(* Logix 5000 AddOnInstructionDefinition export Banner_QS18COD_Param_v4; software revision 33.00 *)

TYPE Banner_IOL_Port_v4 :   // UDT that has all of the data items necessary to communicate with a specific Port on a IO-Link Master
STRUCT
   Port_Controlled : INT;   // Each bit represents a port on an IO-Link Master. Set to 1 to tell AOI to control that port.
   Port_Activate : INT;   // Each bit represents a port on an IO-Link Master. When ON that port will process any commands in queue.
   Port_Read : INT;   // Each bit represents a port on an IO-Link Master. Used to determine when device AOI has requested a Read command.
   Port_Write : INT;   // Each bit represents a port on an IO-Link Master. Used to determine when device AOI has requested a Write command.
   Port_RW_Complete : INT;   // Each bit represents a port on an IO-Link Master. Tells device AOI that Read or Write request has been completed.
   Port_Device_Read : INT;
   Data_Transfer : SINT[190];   // Array to transfer data from IO-Master to device AOIs.
END_STRUCT
END_TYPE

TYPE Banner_QS18COD_RD_v4 :   // UDT that stores the Write Data for a QS18COD.
STRUCT
   Master_Cycle_Time : INT;
   Min_Cycle_Time : INT;
   M_Sequence_Capability : INT;
   IO_Link_Version_ID : INT;
   Process_Data_Input_Length : INT;
   Process_Data_Output_Length : INT;
   Combined_Vendor_ID : DINT;   // IO-Link Vendor ID
   Vendor_ID1 : INT;
   Vendor_ID2 : INT;
   Combined_Device_ID : DINT;   // IO-Link Device ID
   Device_ID1 : INT;
   Device_ID2 : INT;
   Device_ID3 : INT;
   Serial_Number : STRING;
   Quality_of_Health : INT;
   Normalized_Signal_Strength : INT;
   Quality_of_Teach : INT;
   Health_Lower_Limit : INT;
   Health_Upper_Limit : INT;
   Lower_Sensing_Threshold : INT;
   Upper_Sensing_Threshold : INT;
   Sensor_Operationl_Mode : INT;
END_STRUCT
END_TYPE

TYPE Banner_QS18COD_v4 :   // All of the parameters for a QS18COD.
STRUCT
   Initial_Global_Read : BOOL;   // Determines if all of the IO-Link data has been read into the PLC yet
   Command : INT;   // Value placed in here will activate a read or write to a specifc IO-Link Index
   Read_Data : Banner_QS18COD_RD_v4;   // Read Only Data
   Write_Data : Banner_QS18COD_WD_v4;   // Write Data
   Archive : Banner_QS18COD_WD_v4;   // Archive Data
   Reset : BOOL;   // Resets AOI. This will force a complete parameter read of the sensor.
END_STRUCT
END_TYPE

TYPE Banner_QS18COD_WD_v4 :   // UDT that stores the Write Data for a QS18COD.
STRUCT
   System_Command : INT;   // See IODD file for list of commands that can be activated via the System Command interface
   Parameter_Access_Lock : SINT;   // Write access to all parameters is prohibited while value is 1. Only this parameter can be adjusted when value is 1.
   Data_Storage_Lock : SINT;   // Automatic data storage is disabled when this value is equal to 1. Read access is not affected.
   Local_Parameterization_Lock : SINT;   // Parameterization via local control elements on device is disabled.
   Local_User_Interface_Lock : SINT;   // Operation of local user interface is disabled.
   BDC1_Switchpoint_Logic : INT;   // 0 = Light Operate, 1 = Dark Operate
   BDC1_BDC_Mode : INT;   // 1 = 1-Pt BGS, 128 = 2-Pt, 129 = Dynamic, 130 = Window or FGS, 131 = Dual
   BDC1_Hysteresis : DINT;   // Should always be 0
   User_Health_Setting : INT;   // 0 to 90
   Health_Mode : INT;   // 0=Auto, 1=User
   Threshold_Offset : INT;   // 0=8, 1=16, 2=32. Controls the Sensitivity of the Sensor.
   Auto_Compensaton : INT;   // 0=Disabled, 1=Enabled
   Delay_Timer_2 : DINT;   // 0 to 90000 ms
   Delay_Timer_1 : DINT;   // 0 to 90000 ms
   Delay_Mode : INT;   // 0=Disabled, 1=On Off Delay, 2=On One Shot, 3=Off One Shot
   Pin_2_Configuration : SINT;   // 0=Deactivated, 1=Emitter Enable, 2=Emitter Disabled, 3=Remote Input, 4=Detection Output, 5=Complimentary Output, 6=Health Output Active, 7=Health Output Inactive
   Polarity_of_Pins_2_and_4 : INT;   // 0 = Push Pull, 1 = PNP, 2 = NPN
END_STRUCT
END_TYPE

ADD_ON_INSTRUCTION Banner_QS18COD_Param_v4   (* revision 4.0, vendor Banner Engineering *)
// AOI to read and write parameter data to an IO-Link QS18 COD.
VAR_IN_OUT
   QS18COD : Banner_QS18COD_v4; {required}
   Port_Data : Banner_IOL_Port_v4; {required}
END_VAR
VAR_INPUT
   Port : DINT; {required}
END_VAR
VAR
   Local_Control : DINT; {access None}
   Global_Read_Command_Value : INT; {access None}
   Global_Write_Command_Value : INT; {access None}
   Command_Being_Processed : BOOL; {access None}
   Update_Archive : BOOL; {access None}
   Index_Write_Inprocess : INT; {access None}
   Index_Write_Control : INT; {access None}
   Inprocess_Index : DINT; {access None}
END_VAR

ROUTINE Logic   (* ladder *)
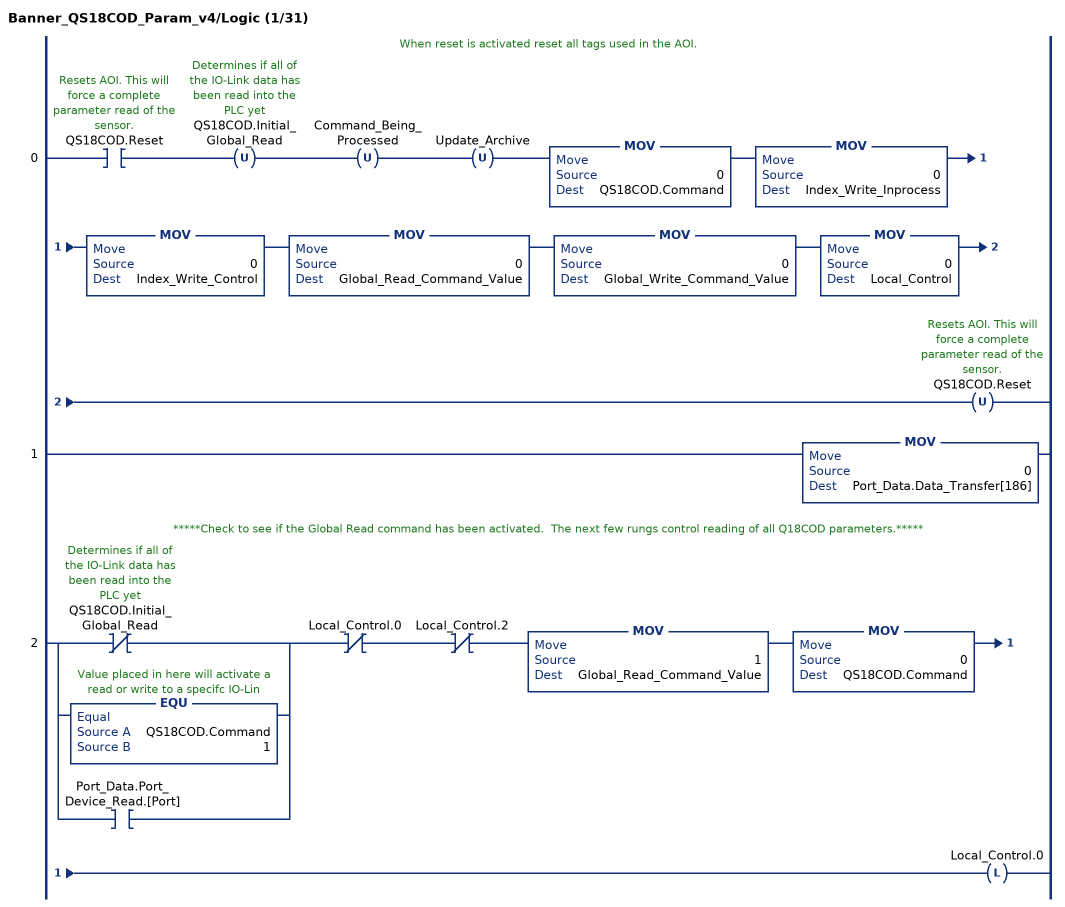
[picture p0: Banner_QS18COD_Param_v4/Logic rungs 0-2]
   // When reset is activated reset all tags used in the AOI.
   0: XIC(QS18COD.Reset)OTU(QS18COD.Initial_Global_Read)OTU(Command_Being_Processed)OTU(Update_Archive)MOV(0,QS18COD.Command)MOV(0,Index_Write_Inprocess)MOV(0,Index_Write_Control)MOV(0,Global_Read_Command_Value)MOV(0,Global_Write_Command_Value)MOV(0,Local_Control)OTU(QS18COD.Reset);
   1: MOV(0,Port_Data.Data_Transfer[186]);
   // *****Check to see if the Global Read command has been activated.  The next few rungs control reading of all Q18COD parameters.*****
   2: [XIO(QS18COD.Initial_Global_Read) ,EQU(QS18COD.Command,1) ,XIC(Port_Data.Port_Device_Read.[Port]) ]XIO(Local_Control.0)XIO(Local_Control.2)MOV(1,Global_Read_Command_Value)MOV(0,QS18COD.Command)OTL(Local_Control.0);
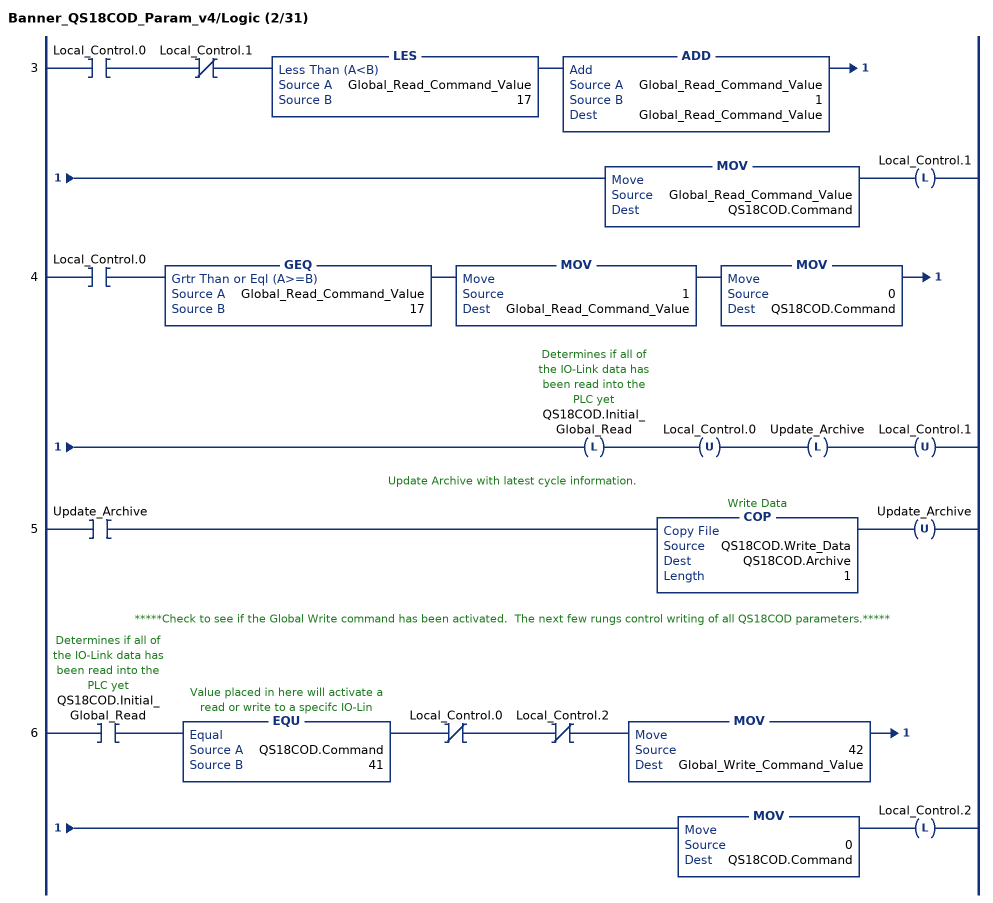
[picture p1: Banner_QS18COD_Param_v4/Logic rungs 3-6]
   3: XIC(Local_Control.0)XIO(Local_Control.1)LES(Global_Read_Command_Value,17)ADD(Global_Read_Command_Value,1,Global_Read_Command_Value)MOV(Global_Read_Command_Value,QS18COD.Command)OTL(Local_Control.1);
   4: XIC(Local_Control.0)GEQ(Global_Read_Command_Value,17)MOV(1,Global_Read_Command_Value)MOV(0,QS18COD.Command)OTL(QS18COD.Initial_Global_Read)OTU(Local_Control.0)OTL(Update_Archive)OTU(Local_Control.1);
   // Update Archive with latest cycle information.
   5: XIC(Update_Archive)COP(QS18COD.Write_Data,QS18COD.Archive,1)OTU(Update_Archive);
   // *****Check to see if the Global Write command has been activated.  The next few rungs control writing of all QS18COD parameters.*****
   6: XIC(QS18COD.Initial_Global_Read)EQU(QS18COD.Command,41)XIO(Local_Control.0)XIO(Local_Control.2)MOV(42,Global_Write_Command_Value)MOV(0,QS18COD.Command)OTL(Local_Control.2);
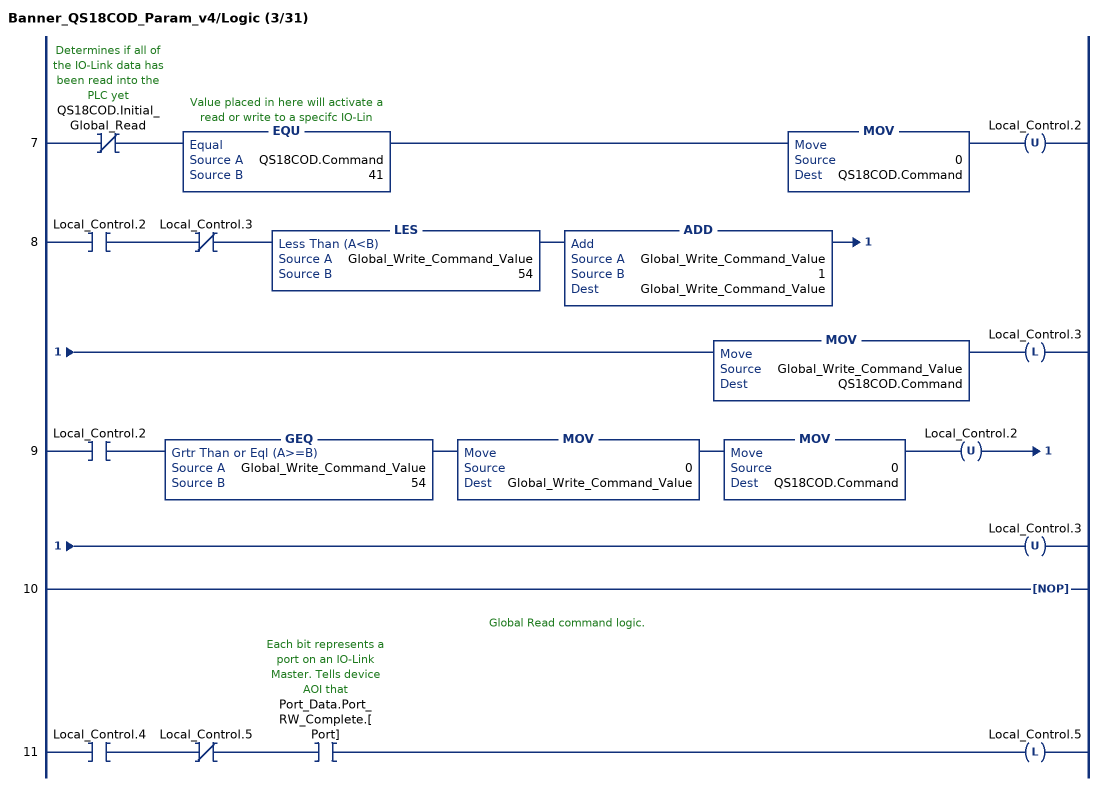
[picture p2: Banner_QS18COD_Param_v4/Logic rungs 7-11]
   7: XIO(QS18COD.Initial_Global_Read)EQU(QS18COD.Command,41)MOV(0,QS18COD.Command)OTU(Local_Control.2);
   8: XIC(Local_Control.2)XIO(Local_Control.3)LES(Global_Write_Command_Value,54)ADD(Global_Write_Command_Value,1,Global_Write_Command_Value)MOV(Global_Write_Command_Value,QS18COD.Command)OTL(Local_Control.3);
   9: XIC(Local_Control.2)GEQ(Global_Write_Command_Value,54)MOV(0,Global_Write_Command_Value)MOV(0,QS18COD.Command)OTU(Local_Control.2)OTU(Local_Control.3);
   10: NOP();
   // Global Read command logic.
   11: XIC(Local_Control.4)XIO(Local_Control.5)XIC(Port_Data.Port_RW_Complete.[Port])OTL(Local_Control.5);
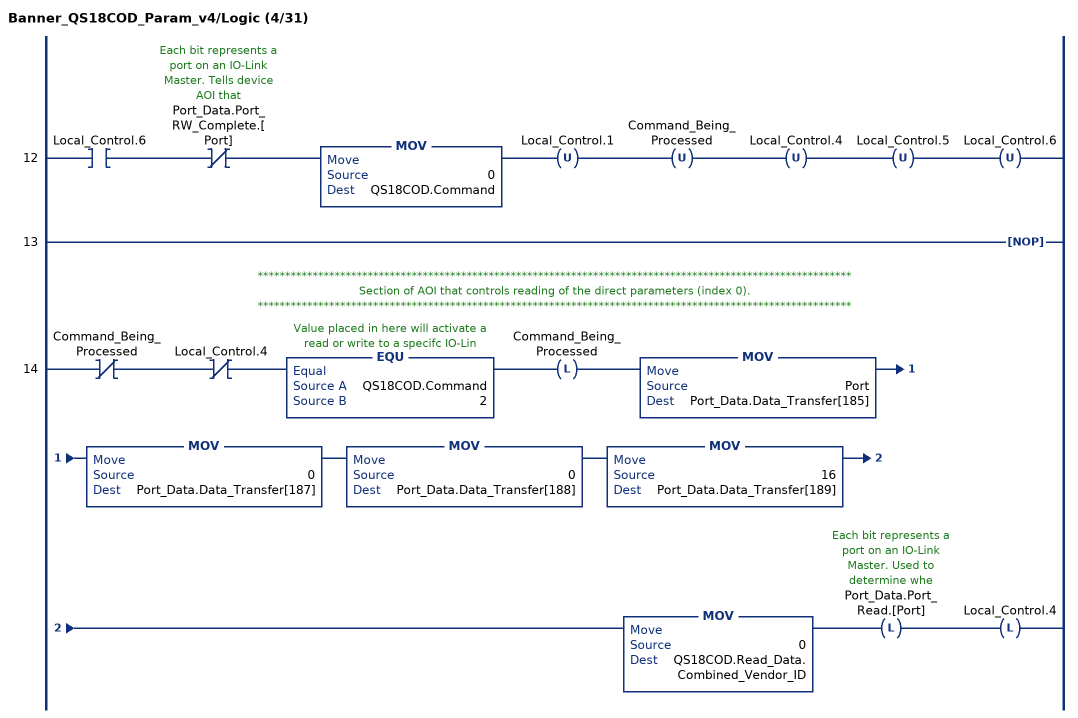
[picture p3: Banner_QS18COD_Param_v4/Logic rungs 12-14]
   12: XIC(Local_Control.6)XIO(Port_Data.Port_RW_Complete.[Port])MOV(0,QS18COD.Command)OTU(Local_Control.1)OTU(Command_Being_Processed)OTU(Local_Control.4)OTU(Local_Control.5)OTU(Local_Control.6);
   13: NOP();
   // ************************************************************************************************************
   // Section of AOI that controls reading of the direct parameters (index 0).
   // ************************************************************************************************************
   14: XIO(Command_Being_Processed)XIO(Local_Control.4)EQU(QS18COD.Command,2)OTL(Command_Being_Processed)MOV(Port,Port_Data.Data_Transfer[185])MOV(0,Port_Data.Data_Transfer[187])MOV(0,Port_Data.Data_Transfer[188])MOV(16,Port_Data.Data_Transfer[189])MOV(0,QS18COD.Read_Data.Combined_Vendor_ID)OTL(Port_Data.Port_Read.[Port])OTL(Local_Control.4);
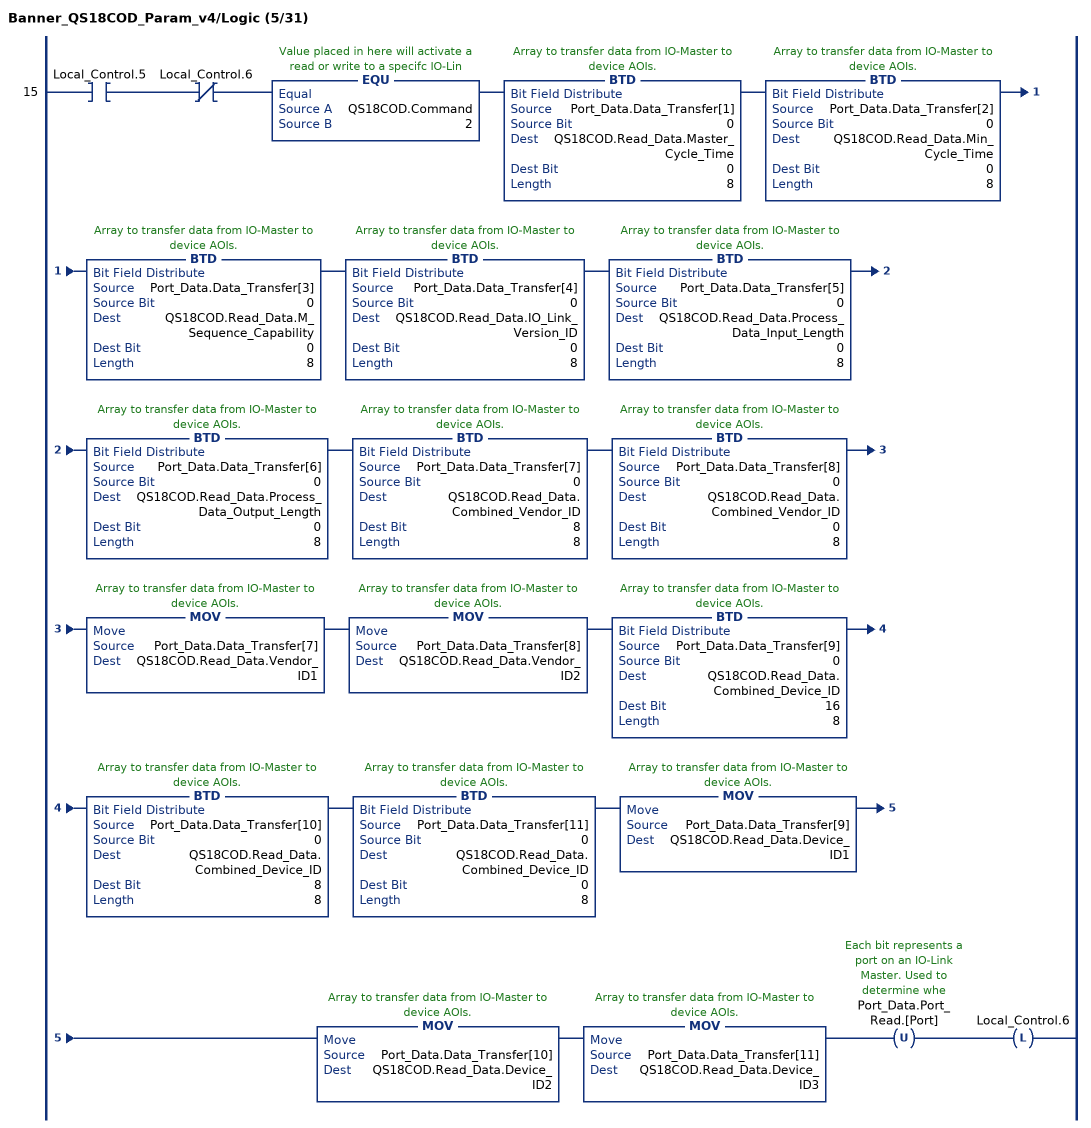
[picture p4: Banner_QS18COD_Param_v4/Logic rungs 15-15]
   15: XIC(Local_Control.5)XIO(Local_Control.6)EQU(QS18COD.Command,2)BTD(Port_Data.Data_Transfer[1],0,QS18COD.Read_Data.Master_Cycle_Time,0,8)BTD(Port_Data.Data_Transfer[2],0,QS18COD.Read_Data.Min_Cycle_Time,0,8)BTD(Port_Data.Data_Transfer[3],0,QS18COD.Read_Data.M_Sequence_Capability,0,8)BTD(Port_Data.Data_Transfer[4],0,QS18COD.Read_Data.IO_Link_Version_ID,0,8)BTD(Port_Data.Data_Transfer[5],0,QS18COD.Read_Data.Process_Data_Input_Length,0,8)BTD(Port_Data.Data_Transfer[6],0,QS18COD.Read_Data.Process_Data_Output_Length,0,8)BTD(Port_Data.Data_Transfer[7],0,QS18COD.Read_Data.Combined_Vendor_ID,8,8)BTD(Port_Data.Data_Transfer[8],0,QS18COD.Read_Data.Combined_Vendor_ID,0,8)MOV(Port_Data.Data_Transfer[7],QS18COD.Read_Data.Vendor_ID1)MOV(Port_Data.Data_Transfer[8],QS18COD.Read_Data.Vendor_ID2)BTD(Port_Data.Data_Transfer[9],0,QS18COD.Read_Data.Combined_Device_ID,16,8)BTD(Port_Data.Data_Transfer[10],0,QS18COD.Read_Data.Combined_Device_ID,8,8)BTD(Port_Data.Data_Transfer[11],0,QS18COD.Read_Data.Combined_Device_ID,0,8)MOV(Port_Data.Data_Transfer[9],QS18COD.Read_Data.Device_ID1)MOV(Port_Data.Data_Transfer[10],QS18COD.Read_Data.Device_ID2)MOV(Port_Data.Data_Transfer[11],QS18COD.Read_Data.Device_ID3)OTU(Port_Data.Port_Read.[Port])OTL(Local_Control.6);
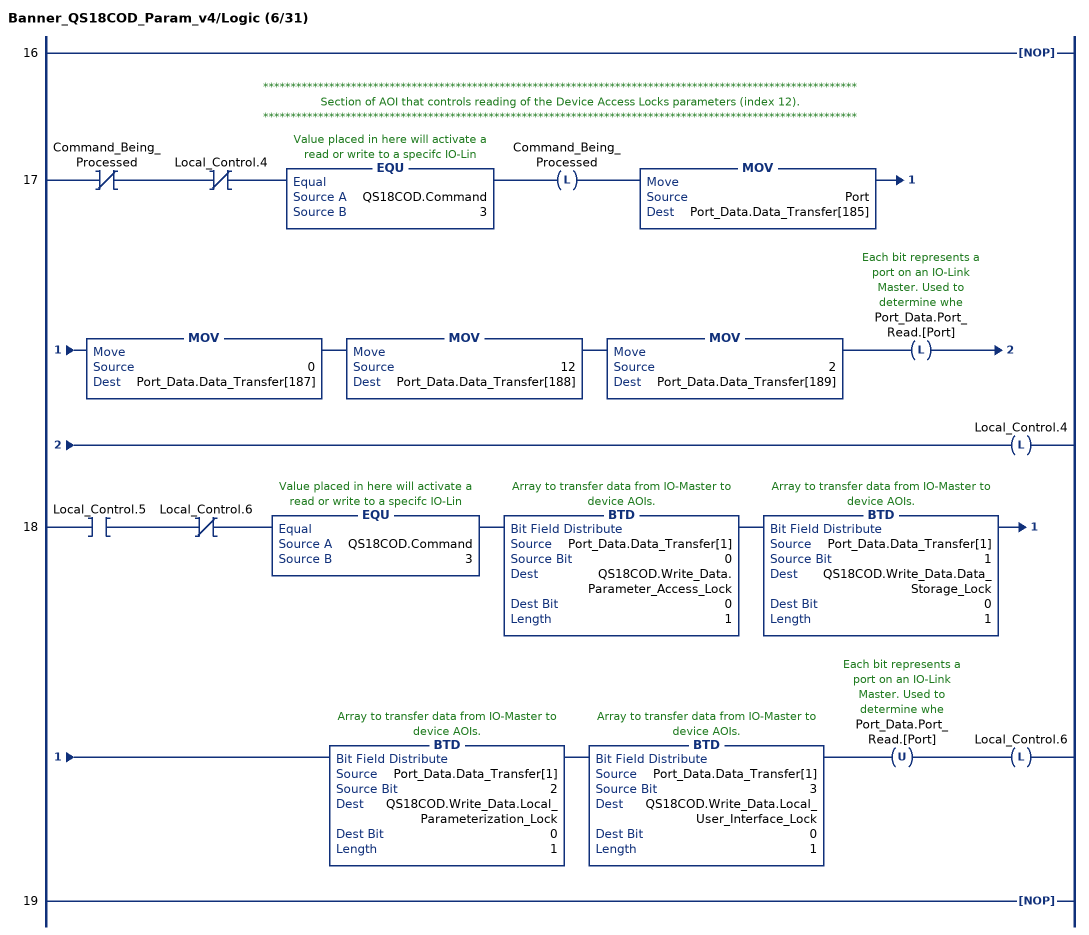
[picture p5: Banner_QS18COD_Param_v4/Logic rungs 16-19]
   16: NOP();
   // ************************************************************************************************************
   // Section of AOI that controls reading of the Device Access Locks parameters (index 12).
   // ************************************************************************************************************
   17: XIO(Command_Being_Processed)XIO(Local_Control.4)EQU(QS18COD.Command,3)OTL(Command_Being_Processed)MOV(Port,Port_Data.Data_Transfer[185])MOV(0,Port_Data.Data_Transfer[187])MOV(12,Port_Data.Data_Transfer[188])MOV(2,Port_Data.Data_Transfer[189])OTL(Port_Data.Port_Read.[Port])OTL(Local_Control.4);
   18: XIC(Local_Control.5)XIO(Local_Control.6)EQU(QS18COD.Command,3)BTD(Port_Data.Data_Transfer[1],0,QS18COD.Write_Data.Parameter_Access_Lock,0,1)BTD(Port_Data.Data_Transfer[1],1,QS18COD.Write_Data.Data_Storage_Lock,0,1)BTD(Port_Data.Data_Transfer[1],2,QS18COD.Write_Data.Local_Parameterization_Lock,0,1)BTD(Port_Data.Data_Transfer[1],3,QS18COD.Write_Data.Local_User_Interface_Lock,0,1)OTU(Port_Data.Port_Read.[Port])OTL(Local_Control.6);
   19: NOP();
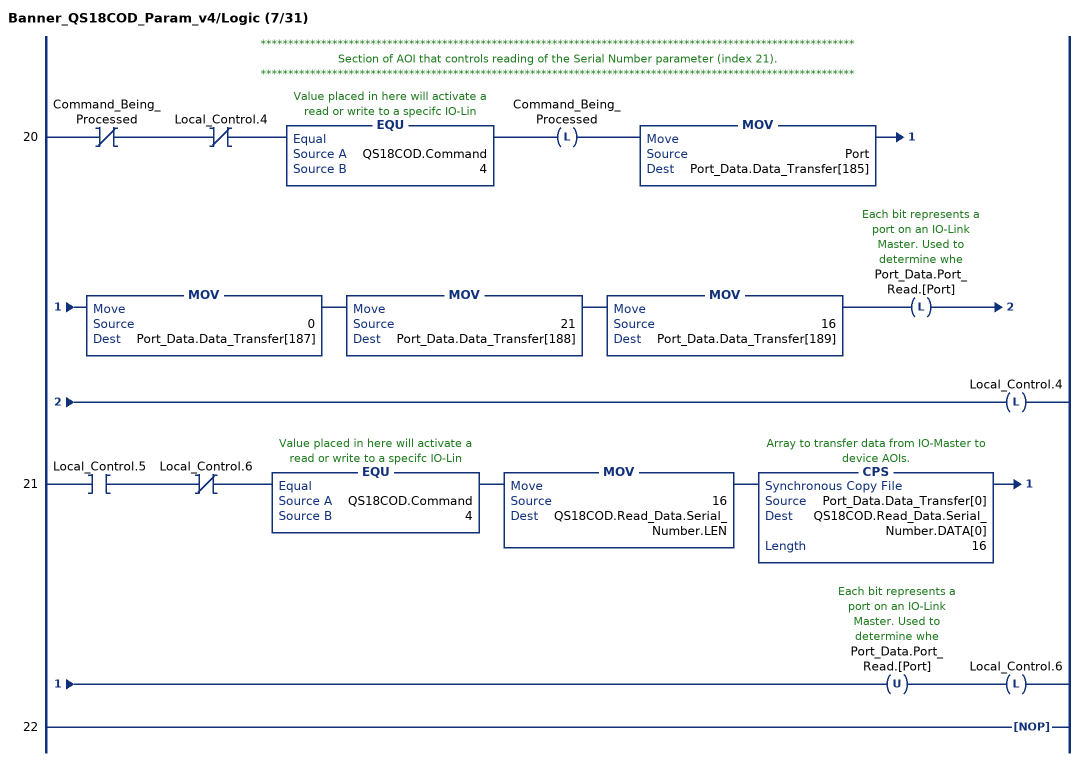
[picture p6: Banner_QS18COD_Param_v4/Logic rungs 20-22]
   // ************************************************************************************************************
   // Section of AOI that controls reading of the Serial Number parameter (index 21).
   // ************************************************************************************************************
   20: XIO(Command_Being_Processed)XIO(Local_Control.4)EQU(QS18COD.Command,4)OTL(Command_Being_Processed)MOV(Port,Port_Data.Data_Transfer[185])MOV(0,Port_Data.Data_Transfer[187])MOV(21,Port_Data.Data_Transfer[188])MOV(16,Port_Data.Data_Transfer[189])OTL(Port_Data.Port_Read.[Port])OTL(Local_Control.4);
   21: XIC(Local_Control.5)XIO(Local_Control.6)EQU(QS18COD.Command,4)MOV(16,QS18COD.Read_Data.Serial_Number.LEN)CPS(Port_Data.Data_Transfer[0],QS18COD.Read_Data.Serial_Number.DATA[0],16)OTU(Port_Data.Port_Read.[Port])OTL(Local_Control.6);
   22: NOP();
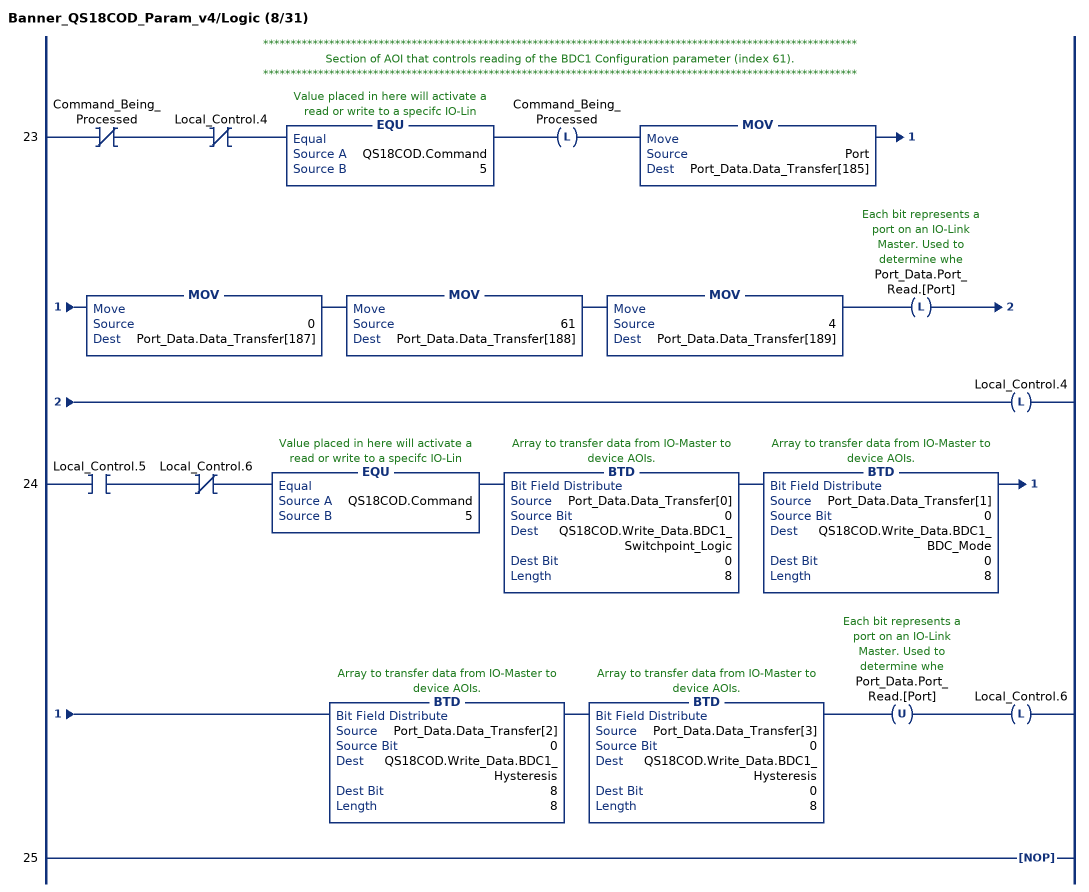
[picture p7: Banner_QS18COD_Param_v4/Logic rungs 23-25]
   // ************************************************************************************************************
   // Section of AOI that controls reading of the BDC1 Configuration parameter (index 61).
   // ************************************************************************************************************
   23: XIO(Command_Being_Processed)XIO(Local_Control.4)EQU(QS18COD.Command,5)OTL(Command_Being_Processed)MOV(Port,Port_Data.Data_Transfer[185])MOV(0,Port_Data.Data_Transfer[187])MOV(61,Port_Data.Data_Transfer[188])MOV(4,Port_Data.Data_Transfer[189])OTL(Port_Data.Port_Read.[Port])OTL(Local_Control.4);
   24: XIC(Local_Control.5)XIO(Local_Control.6)EQU(QS18COD.Command,5)BTD(Port_Data.Data_Transfer[0],0,QS18COD.Write_Data.BDC1_Switchpoint_Logic,0,8)BTD(Port_Data.Data_Transfer[1],0,QS18COD.Write_Data.BDC1_BDC_Mode,0,8)BTD(Port_Data.Data_Transfer[2],0,QS18COD.Write_Data.BDC1_Hysteresis,8,8)BTD(Port_Data.Data_Transfer[3],0,QS18COD.Write_Data.BDC1_Hysteresis,0,8)OTU(Port_Data.Port_Read.[Port])OTL(Local_Control.6);
   25: NOP();
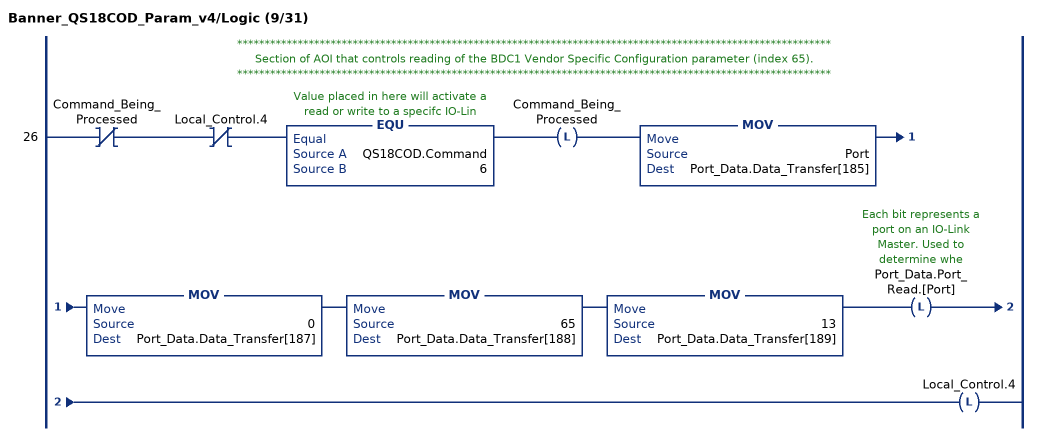
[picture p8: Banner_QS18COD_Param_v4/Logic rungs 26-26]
   // ************************************************************************************************************
   // Section of AOI that controls reading of the BDC1 Vendor Specific Configuration parameter (index 65).
   // ************************************************************************************************************
   26: XIO(Command_Being_Processed)XIO(Local_Control.4)EQU(QS18COD.Command,6)OTL(Command_Being_Processed)MOV(Port,Port_Data.Data_Transfer[185])MOV(0,Port_Data.Data_Transfer[187])MOV(65,Port_Data.Data_Transfer[188])MOV(13,Port_Data.Data_Transfer[189])OTL(Port_Data.Port_Read.[Port])OTL(Local_Control.4);
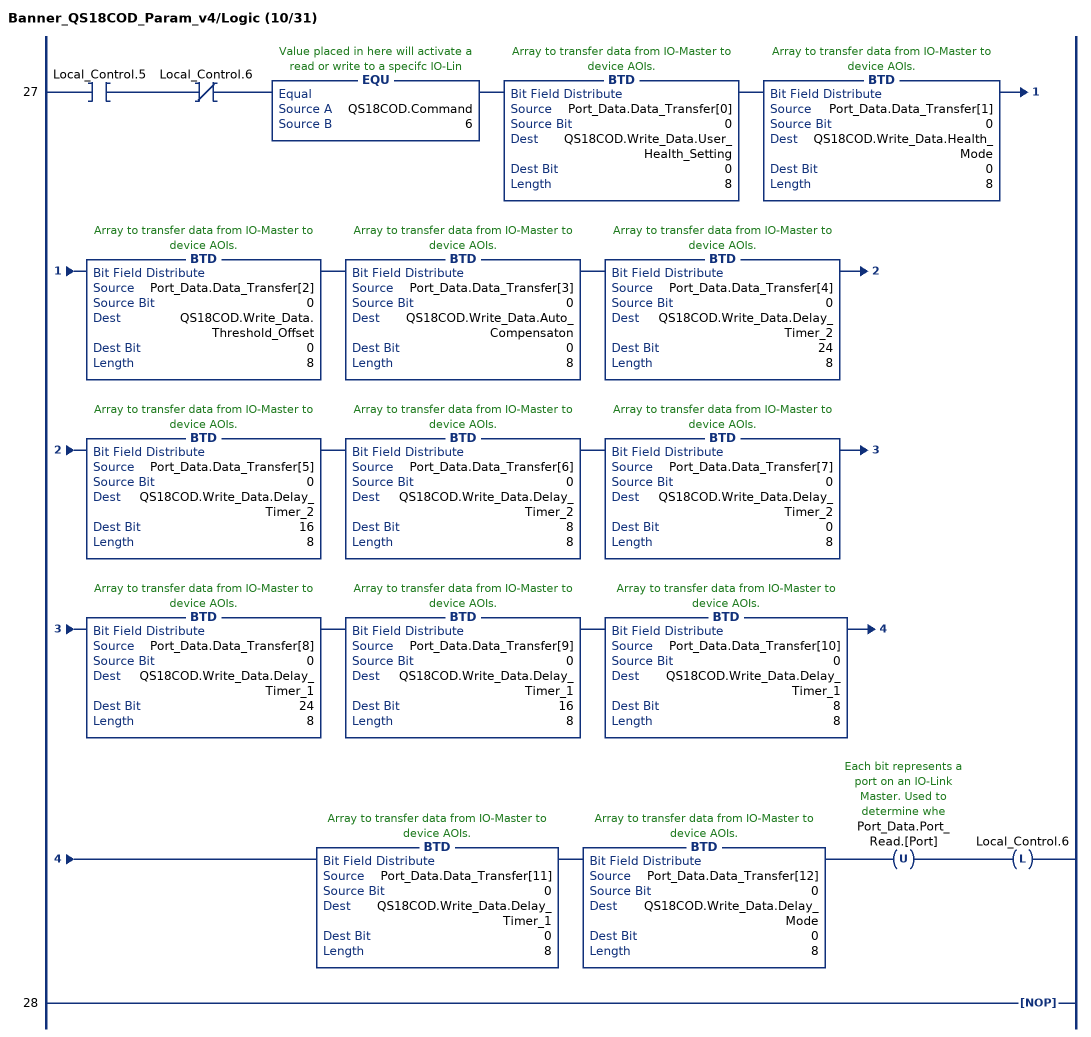
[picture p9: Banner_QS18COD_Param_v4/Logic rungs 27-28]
   27: XIC(Local_Control.5)XIO(Local_Control.6)EQU(QS18COD.Command,6)BTD(Port_Data.Data_Transfer[0],0,QS18COD.Write_Data.User_Health_Setting,0,8)BTD(Port_Data.Data_Transfer[1],0,QS18COD.Write_Data.Health_Mode,0,8)BTD(Port_Data.Data_Transfer[2],0,QS18COD.Write_Data.Threshold_Offset,0,8)BTD(Port_Data.Data_Transfer[3],0,QS18COD.Write_Data.Auto_Compensaton,0,8)BTD(Port_Data.Data_Transfer[4],0,QS18COD.Write_Data.Delay_Timer_2,24,8)BTD(Port_Data.Data_Transfer[5],0,QS18COD.Write_Data.Delay_Timer_2,16,8)BTD(Port_Data.Data_Transfer[6],0,QS18COD.Write_Data.Delay_Timer_2,8,8)BTD(Port_Data.Data_Transfer[7],0,QS18COD.Write_Data.Delay_Timer_2,0,8)BTD(Port_Data.Data_Transfer[8],0,QS18COD.Write_Data.Delay_Timer_1,24,8)BTD(Port_Data.Data_Transfer[9],0,QS18COD.Write_Data.Delay_Timer_1,16,8)BTD(Port_Data.Data_Transfer[10],0,QS18COD.Write_Data.Delay_Timer_1,8,8)BTD(Port_Data.Data_Transfer[11],0,QS18COD.Write_Data.Delay_Timer_1,0,8)BTD(Port_Data.Data_Transfer[12],0,QS18COD.Write_Data.Delay_Mode,0,8)OTU(Port_Data.Port_Read.[Port])OTL(Local_Control.6);
   28: NOP();
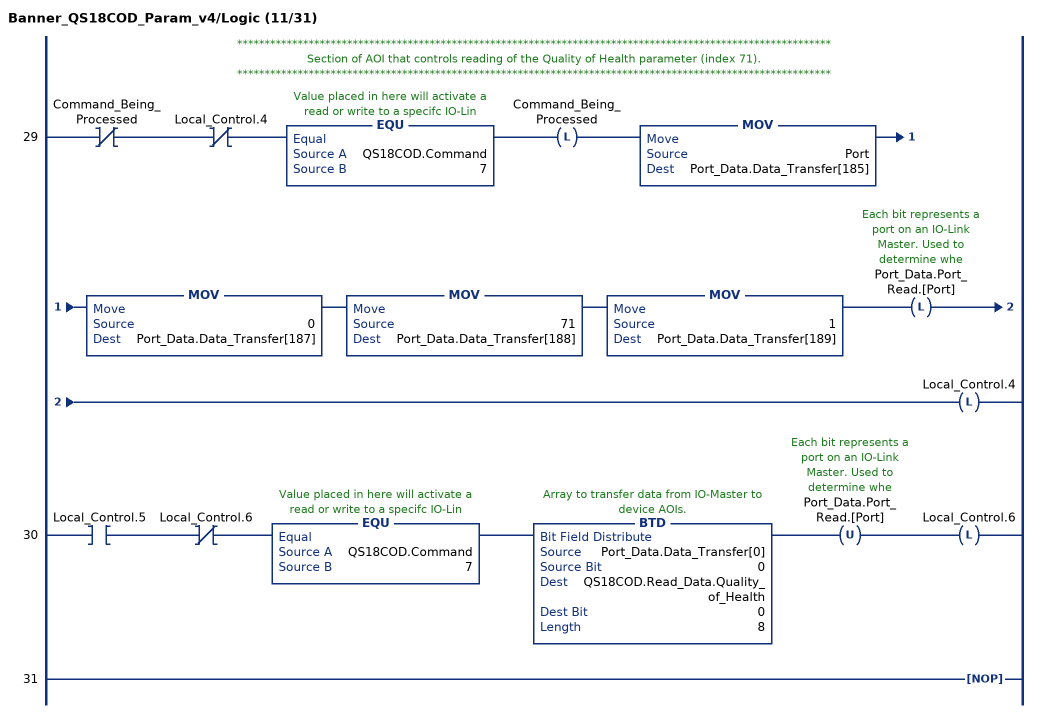
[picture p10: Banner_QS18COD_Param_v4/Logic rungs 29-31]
   // ************************************************************************************************************
   // Section of AOI that controls reading of the Quality of Health parameter (index 71).
   // ************************************************************************************************************
   29: XIO(Command_Being_Processed)XIO(Local_Control.4)EQU(QS18COD.Command,7)OTL(Command_Being_Processed)MOV(Port,Port_Data.Data_Transfer[185])MOV(0,Port_Data.Data_Transfer[187])MOV(71,Port_Data.Data_Transfer[188])MOV(1,Port_Data.Data_Transfer[189])OTL(Port_Data.Port_Read.[Port])OTL(Local_Control.4);
   30: XIC(Local_Control.5)XIO(Local_Control.6)EQU(QS18COD.Command,7)BTD(Port_Data.Data_Transfer[0],0,QS18COD.Read_Data.Quality_of_Health,0,8)OTU(Port_Data.Port_Read.[Port])OTL(Local_Control.6);
   31: NOP();
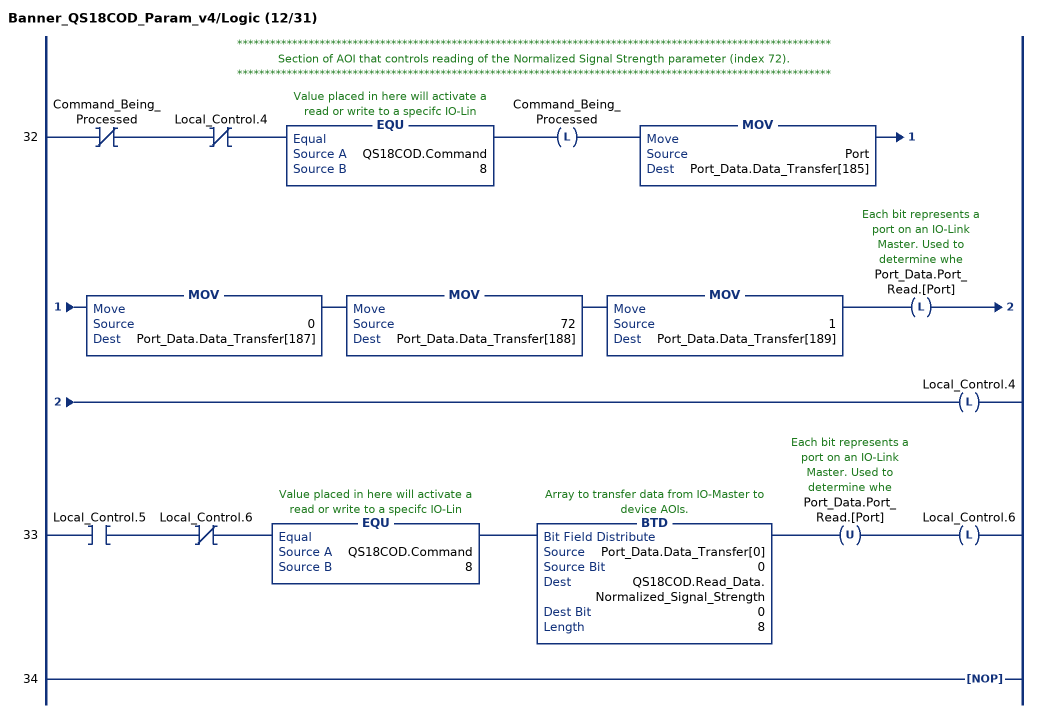
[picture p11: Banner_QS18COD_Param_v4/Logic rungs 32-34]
   // ************************************************************************************************************
   // Section of AOI that controls reading of the Normalized Signal Strength parameter (index 72).
   // ************************************************************************************************************
   32: XIO(Command_Being_Processed)XIO(Local_Control.4)EQU(QS18COD.Command,8)OTL(Command_Being_Processed)MOV(Port,Port_Data.Data_Transfer[185])MOV(0,Port_Data.Data_Transfer[187])MOV(72,Port_Data.Data_Transfer[188])MOV(1,Port_Data.Data_Transfer[189])OTL(Port_Data.Port_Read.[Port])OTL(Local_Control.4);
   33: XIC(Local_Control.5)XIO(Local_Control.6)EQU(QS18COD.Command,8)BTD(Port_Data.Data_Transfer[0],0,QS18COD.Read_Data.Normalized_Signal_Strength,0,8)OTU(Port_Data.Port_Read.[Port])OTL(Local_Control.6);
   34: NOP();
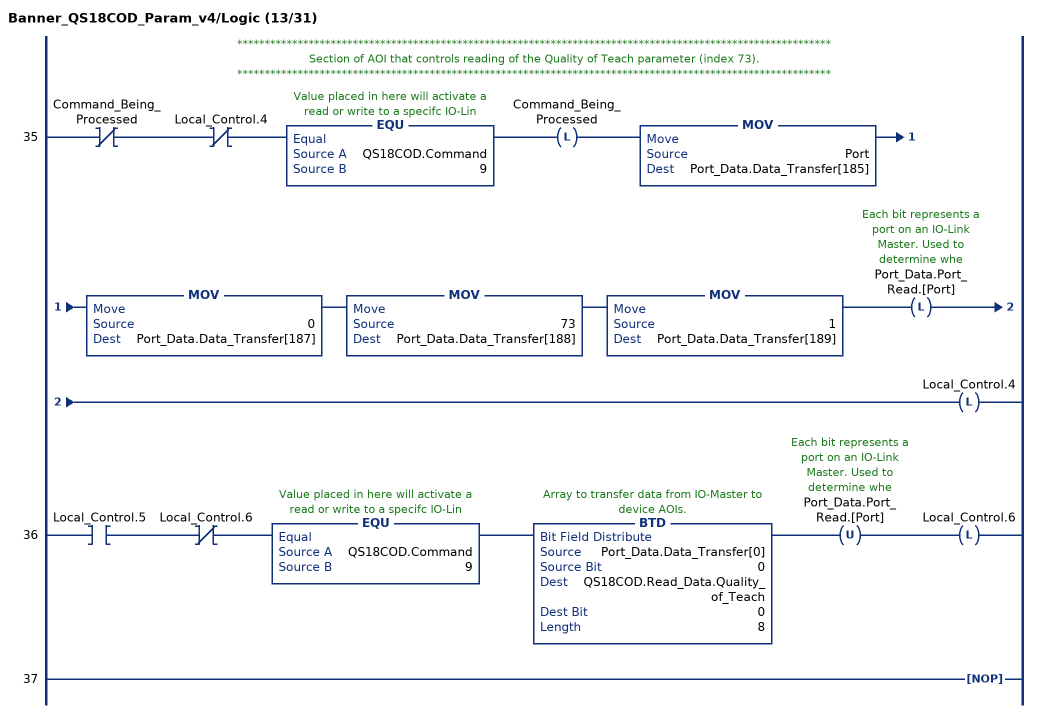
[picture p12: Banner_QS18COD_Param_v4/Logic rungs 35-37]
   // ************************************************************************************************************
   // Section of AOI that controls reading of the Quality of Teach parameter (index 73).
   // ************************************************************************************************************
   35: XIO(Command_Being_Processed)XIO(Local_Control.4)EQU(QS18COD.Command,9)OTL(Command_Being_Processed)MOV(Port,Port_Data.Data_Transfer[185])MOV(0,Port_Data.Data_Transfer[187])MOV(73,Port_Data.Data_Transfer[188])MOV(1,Port_Data.Data_Transfer[189])OTL(Port_Data.Port_Read.[Port])OTL(Local_Control.4);
   36: XIC(Local_Control.5)XIO(Local_Control.6)EQU(QS18COD.Command,9)BTD(Port_Data.Data_Transfer[0],0,QS18COD.Read_Data.Quality_of_Teach,0,8)OTU(Port_Data.Port_Read.[Port])OTL(Local_Control.6);
   37: NOP();
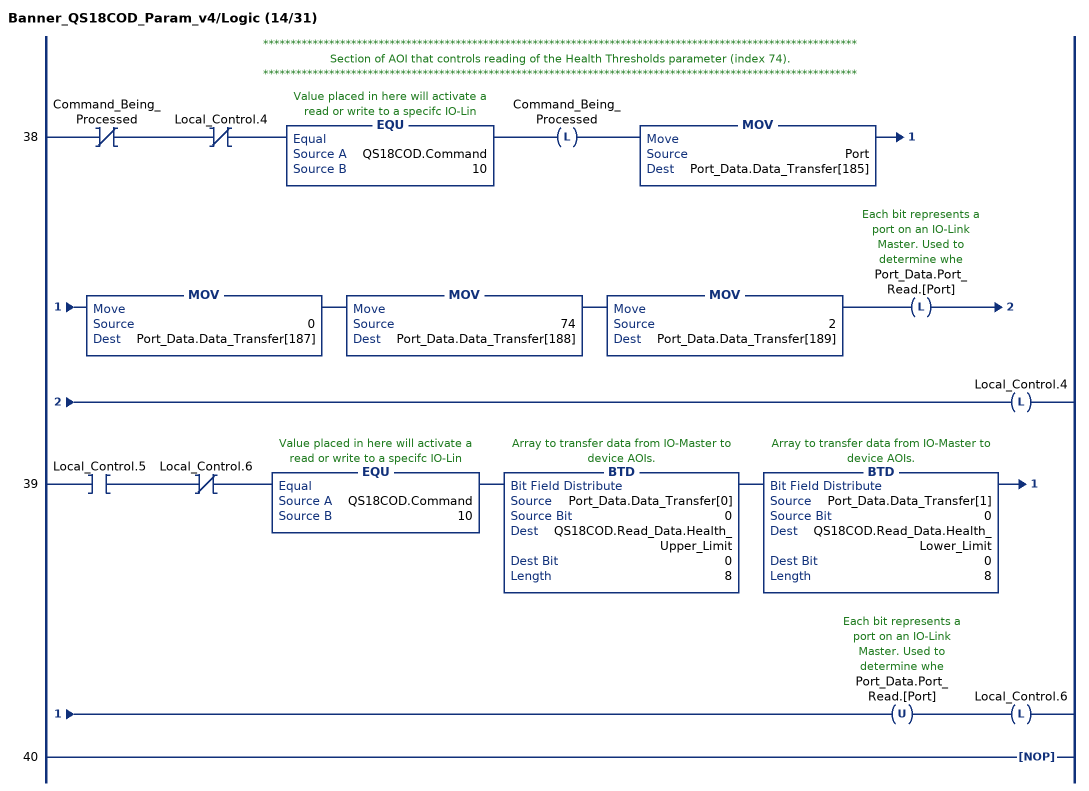
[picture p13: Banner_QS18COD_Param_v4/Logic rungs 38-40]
   // ************************************************************************************************************
   // Section of AOI that controls reading of the Health Thresholds parameter (index 74).
   // ************************************************************************************************************
   38: XIO(Command_Being_Processed)XIO(Local_Control.4)EQU(QS18COD.Command,10)OTL(Command_Being_Processed)MOV(Port,Port_Data.Data_Transfer[185])MOV(0,Port_Data.Data_Transfer[187])MOV(74,Port_Data.Data_Transfer[188])MOV(2,Port_Data.Data_Transfer[189])OTL(Port_Data.Port_Read.[Port])OTL(Local_Control.4);
   39: XIC(Local_Control.5)XIO(Local_Control.6)EQU(QS18COD.Command,10)BTD(Port_Data.Data_Transfer[0],0,QS18COD.Read_Data.Health_Upper_Limit,0,8)BTD(Port_Data.Data_Transfer[1],0,QS18COD.Read_Data.Health_Lower_Limit,0,8)OTU(Port_Data.Port_Read.[Port])OTL(Local_Control.6);
   40: NOP();
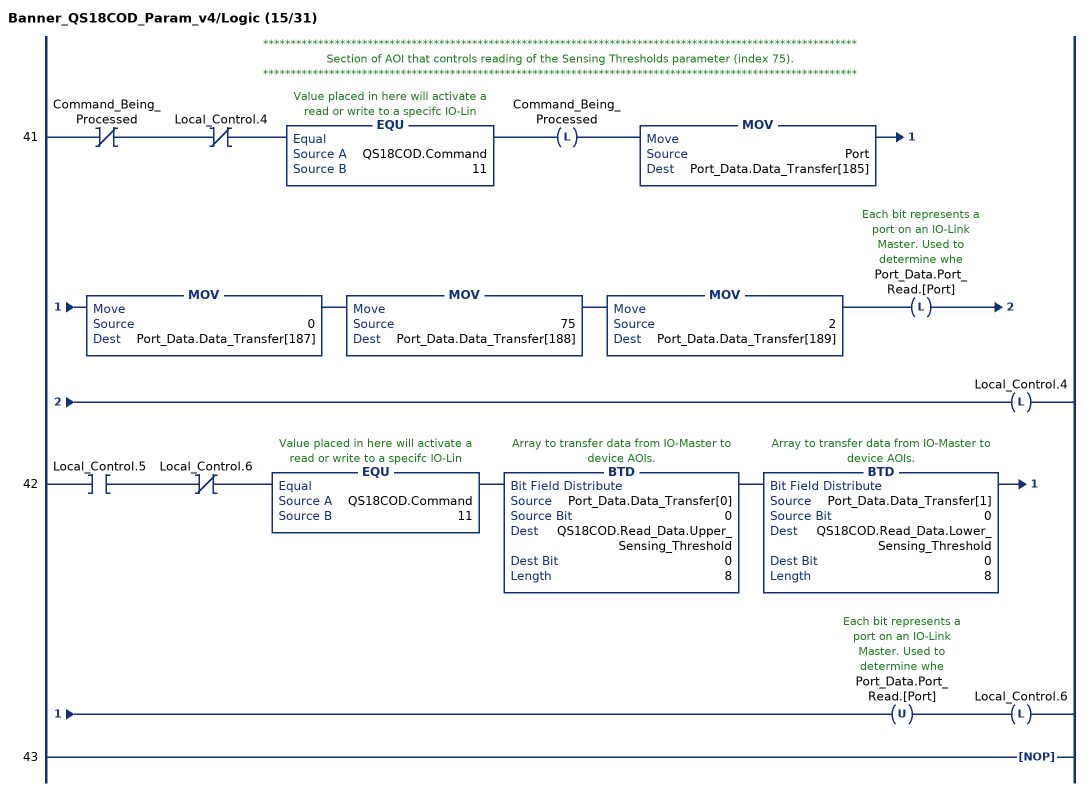
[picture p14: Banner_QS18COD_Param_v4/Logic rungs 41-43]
   // ************************************************************************************************************
   // Section of AOI that controls reading of the Sensing Thresholds parameter (index 75).
   // ************************************************************************************************************
   41: XIO(Command_Being_Processed)XIO(Local_Control.4)EQU(QS18COD.Command,11)OTL(Command_Being_Processed)MOV(Port,Port_Data.Data_Transfer[185])MOV(0,Port_Data.Data_Transfer[187])MOV(75,Port_Data.Data_Transfer[188])MOV(2,Port_Data.Data_Transfer[189])OTL(Port_Data.Port_Read.[Port])OTL(Local_Control.4);
   42: XIC(Local_Control.5)XIO(Local_Control.6)EQU(QS18COD.Command,11)BTD(Port_Data.Data_Transfer[0],0,QS18COD.Read_Data.Upper_Sensing_Threshold,0,8)BTD(Port_Data.Data_Transfer[1],0,QS18COD.Read_Data.Lower_Sensing_Threshold,0,8)OTU(Port_Data.Port_Read.[Port])OTL(Local_Control.6);
   43: NOP();
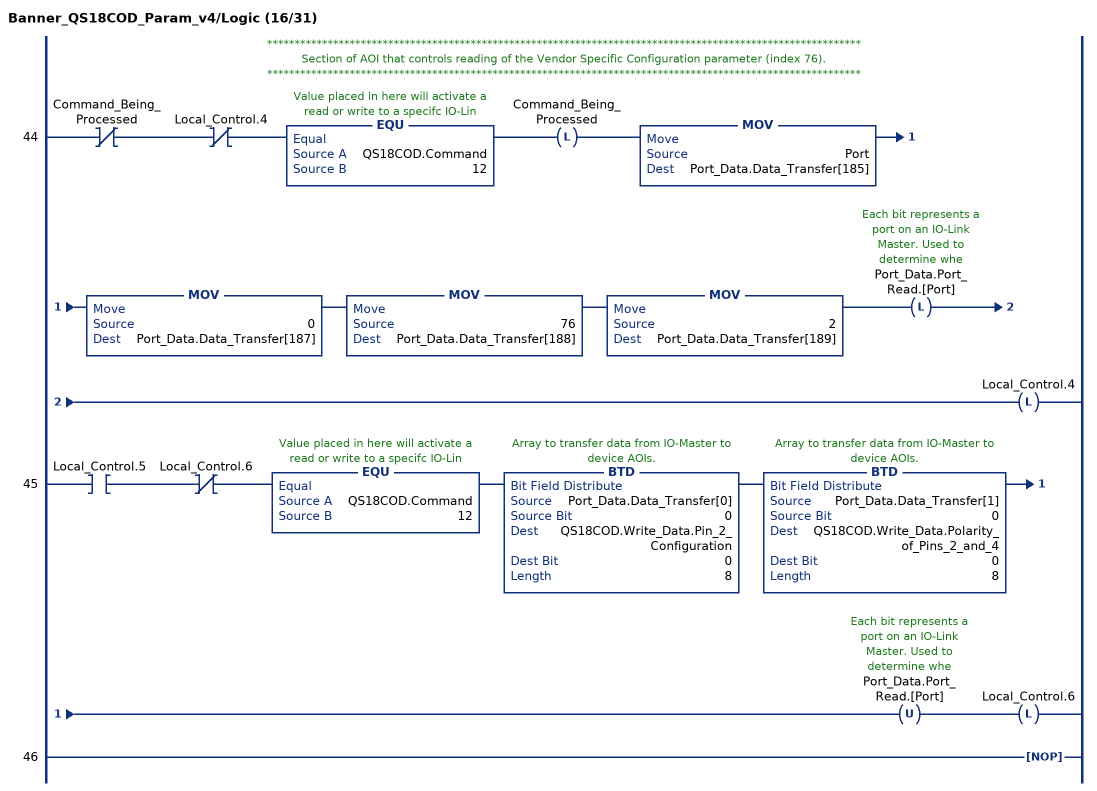
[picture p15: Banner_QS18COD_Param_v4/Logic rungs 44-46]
   // ************************************************************************************************************
   // Section of AOI that controls reading of the Vendor Specific Configuration parameter (index 76).
   // ************************************************************************************************************
   44: XIO(Command_Being_Processed)XIO(Local_Control.4)EQU(QS18COD.Command,12)OTL(Command_Being_Processed)MOV(Port,Port_Data.Data_Transfer[185])MOV(0,Port_Data.Data_Transfer[187])MOV(76,Port_Data.Data_Transfer[188])MOV(2,Port_Data.Data_Transfer[189])OTL(Port_Data.Port_Read.[Port])OTL(Local_Control.4);
   45: XIC(Local_Control.5)XIO(Local_Control.6)EQU(QS18COD.Command,12)BTD(Port_Data.Data_Transfer[0],0,QS18COD.Write_Data.Pin_2_Configuration,0,8)BTD(Port_Data.Data_Transfer[1],0,QS18COD.Write_Data.Polarity_of_Pins_2_and_4,0,8)OTU(Port_Data.Port_Read.[Port])OTL(Local_Control.6);
   46: NOP();
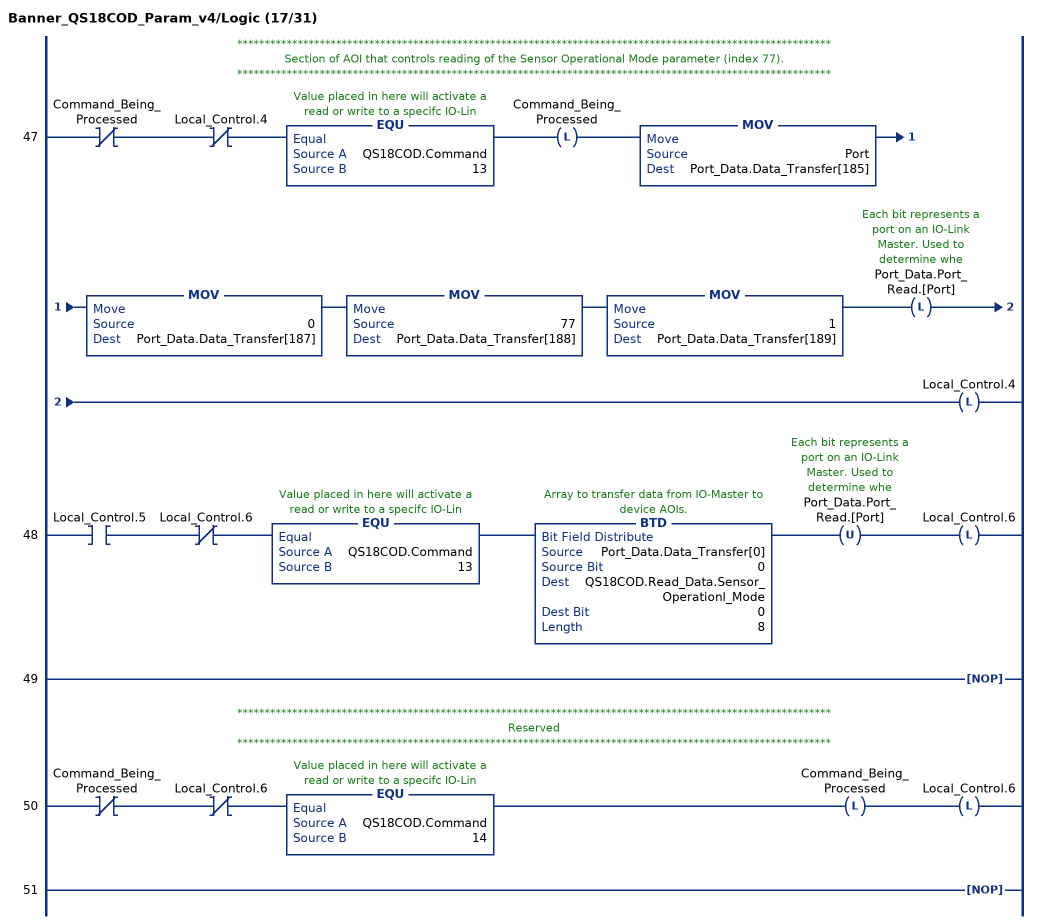
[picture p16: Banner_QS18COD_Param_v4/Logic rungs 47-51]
   // ************************************************************************************************************
   // Section of AOI that controls reading of the Sensor Operational Mode parameter (index 77).
   // ************************************************************************************************************
   47: XIO(Command_Being_Processed)XIO(Local_Control.4)EQU(QS18COD.Command,13)OTL(Command_Being_Processed)MOV(Port,Port_Data.Data_Transfer[185])MOV(0,Port_Data.Data_Transfer[187])MOV(77,Port_Data.Data_Transfer[188])MOV(1,Port_Data.Data_Transfer[189])OTL(Port_Data.Port_Read.[Port])OTL(Local_Control.4);
   48: XIC(Local_Control.5)XIO(Local_Control.6)EQU(QS18COD.Command,13)BTD(Port_Data.Data_Transfer[0],0,QS18COD.Read_Data.Sensor_Operationl_Mode,0,8)OTU(Port_Data.Port_Read.[Port])OTL(Local_Control.6);
   49: NOP();
   // ************************************************************************************************************
   // Reserved
   // ************************************************************************************************************
   50: XIO(Command_Being_Processed)XIO(Local_Control.6)EQU(QS18COD.Command,14)OTL(Command_Being_Processed)OTL(Local_Control.6);
   51: NOP();
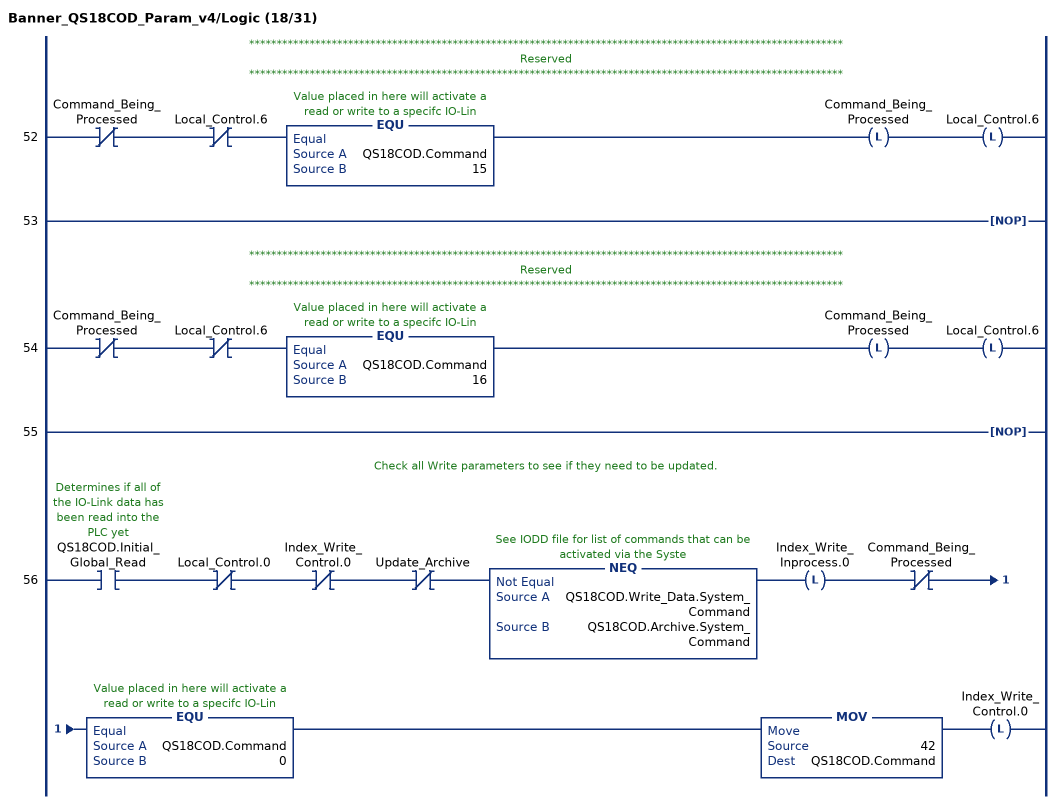
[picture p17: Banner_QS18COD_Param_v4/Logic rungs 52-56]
   // ************************************************************************************************************
   // Reserved
   // ************************************************************************************************************
   52: XIO(Command_Being_Processed)XIO(Local_Control.6)EQU(QS18COD.Command,15)OTL(Command_Being_Processed)OTL(Local_Control.6);
   53: NOP();
   // ************************************************************************************************************
   // Reserved
   // ************************************************************************************************************
   54: XIO(Command_Being_Processed)XIO(Local_Control.6)EQU(QS18COD.Command,16)OTL(Command_Being_Processed)OTL(Local_Control.6);
   55: NOP();
   // Check all Write parameters to see if they need to be updated.
   56: XIC(QS18COD.Initial_Global_Read)XIO(Local_Control.0)XIO(Index_Write_Control.0)XIO(Update_Archive)NEQ(QS18COD.Write_Data.System_Command,QS18COD.Archive.System_Command)OTL(Index_Write_Inprocess.0)XIO(Command_Being_Processed)EQU(QS18COD.Command,0)MOV(42,QS18COD.Command)OTL(Index_Write_Control.0);
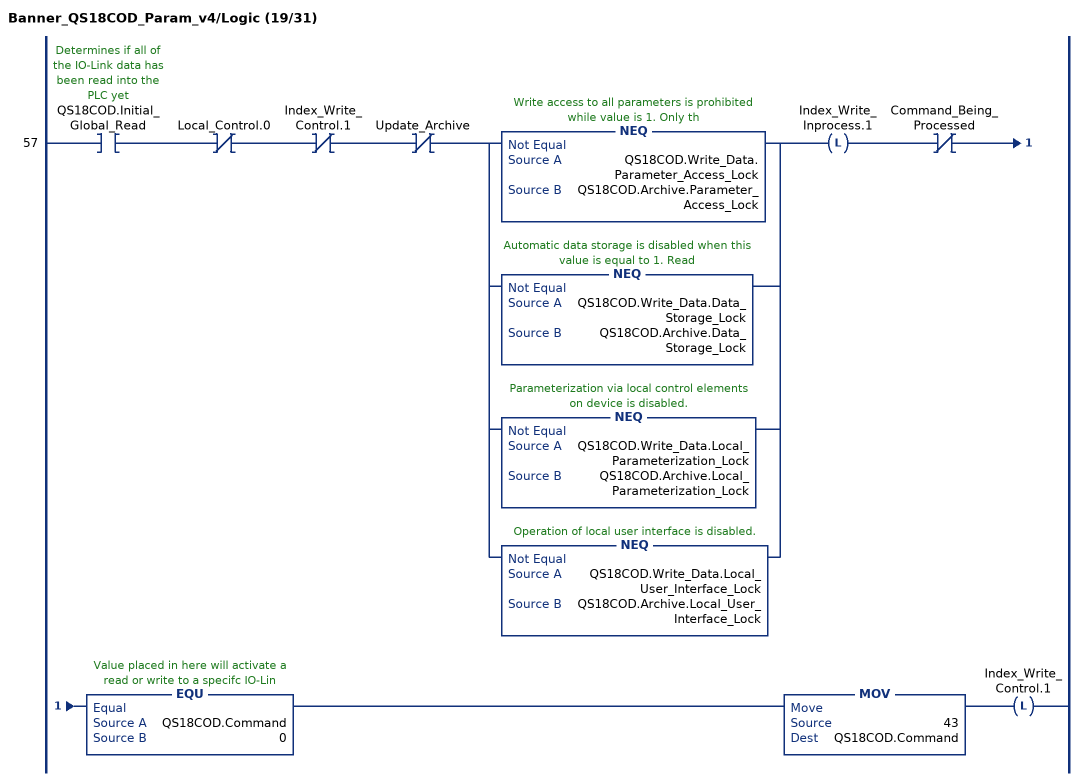
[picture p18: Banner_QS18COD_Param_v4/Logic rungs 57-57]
   57: XIC(QS18COD.Initial_Global_Read)XIO(Local_Control.0)XIO(Index_Write_Control.1)XIO(Update_Archive)[NEQ(QS18COD.Write_Data.Parameter_Access_Lock,QS18COD.Archive.Parameter_Access_Lock) ,NEQ(QS18COD.Write_Data.Data_Storage_Lock,QS18COD.Archive.Data_Storage_Lock) ,NEQ(QS18COD.Write_Data.Local_Parameterization_Lock,QS18COD.Archive.Local_Parameterization_Lock) ,NEQ(QS18COD.Write_Data.Local_User_Interface_Lock,QS18COD.Archive.Local_User_Interface_Lock) ]OTL(Index_Write_Inprocess.1)XIO(Command_Being_Processed)EQU(QS18COD.Command,0)MOV(43,QS18COD.Command)OTL(Index_Write_Control.1);
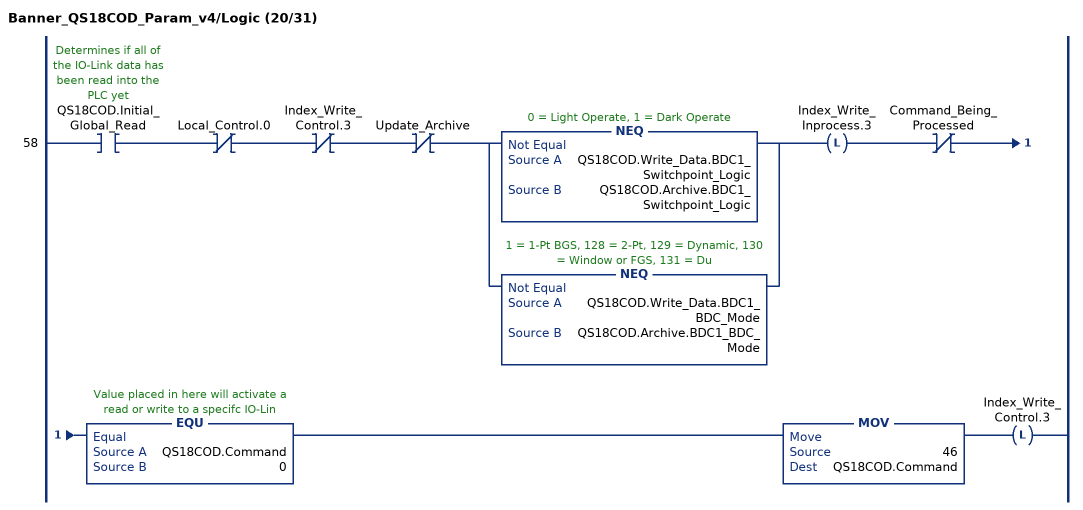
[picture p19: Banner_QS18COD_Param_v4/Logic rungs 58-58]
   58: XIC(QS18COD.Initial_Global_Read)XIO(Local_Control.0)XIO(Index_Write_Control.3)XIO(Update_Archive)[NEQ(QS18COD.Write_Data.BDC1_Switchpoint_Logic,QS18COD.Archive.BDC1_Switchpoint_Logic) ,NEQ(QS18COD.Write_Data.BDC1_BDC_Mode,QS18COD.Archive.BDC1_BDC_Mode) ]OTL(Index_Write_Inprocess.3)XIO(Command_Being_Processed)EQU(QS18COD.Command,0)MOV(46,QS18COD.Command)OTL(Index_Write_Control.3);
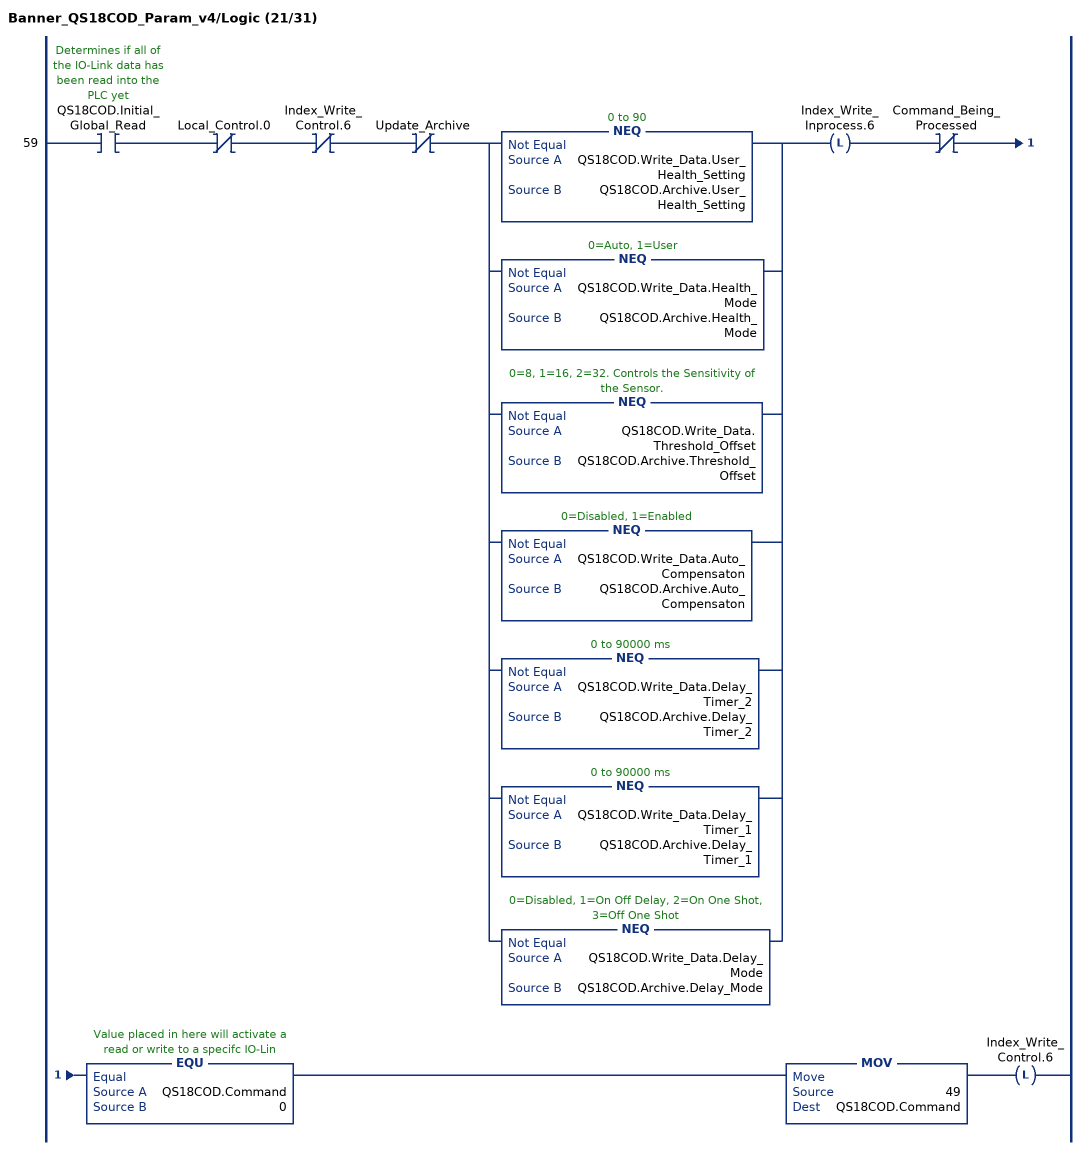
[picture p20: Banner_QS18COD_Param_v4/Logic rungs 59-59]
   59: XIC(QS18COD.Initial_Global_Read)XIO(Local_Control.0)XIO(Index_Write_Control.6)XIO(Update_Archive)[NEQ(QS18COD.Write_Data.User_Health_Setting,QS18COD.Archive.User_Health_Setting) ,NEQ(QS18COD.Write_Data.Health_Mode,QS18COD.Archive.Health_Mode) ,NEQ(QS18COD.Write_Data.Threshold_Offset,QS18COD.Archive.Threshold_Offset) ,NEQ(QS18COD.Write_Data.Auto_Compensaton,QS18COD.Archive.Auto_Compensaton) ,NEQ(QS18COD.Write_Data.Delay_Timer_2,QS18COD.Archive.Delay_Timer_2) ,NEQ(QS18COD.Write_Data.Delay_Timer_1,QS18COD.Archive.Delay_Timer_1) ,NEQ(QS18COD.Write_Data.Delay_Mode,QS18COD.Archive.Delay_Mode) ]OTL(Index_Write_Inprocess.6)XIO(Command_Being_Processed)EQU(QS18COD.Command,0)MOV(49,QS18COD.Command)OTL(Index_Write_Control.6);
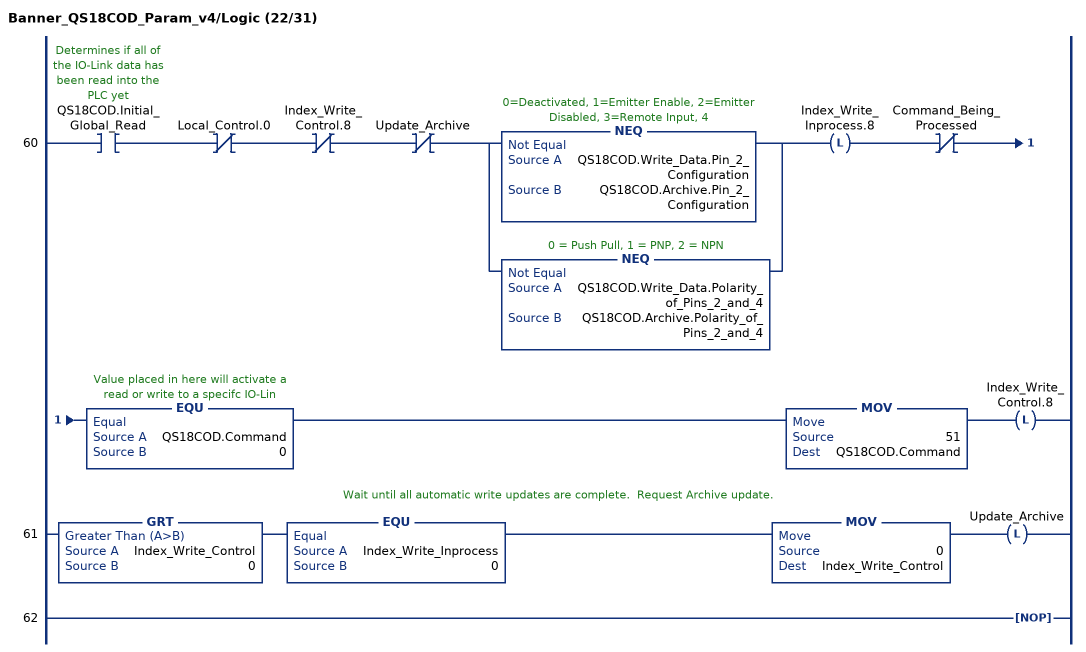
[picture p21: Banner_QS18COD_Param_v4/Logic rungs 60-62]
   60: XIC(QS18COD.Initial_Global_Read)XIO(Local_Control.0)XIO(Index_Write_Control.8)XIO(Update_Archive)[NEQ(QS18COD.Write_Data.Pin_2_Configuration,QS18COD.Archive.Pin_2_Configuration) ,NEQ(QS18COD.Write_Data.Polarity_of_Pins_2_and_4,QS18COD.Archive.Polarity_of_Pins_2_and_4) ]OTL(Index_Write_Inprocess.8)XIO(Command_Being_Processed)EQU(QS18COD.Command,0)MOV(51,QS18COD.Command)OTL(Index_Write_Control.8);
   // Wait until all automatic write updates are complete.  Request Archive update.
   61: GRT(Index_Write_Control,0)EQU(Index_Write_Inprocess,0)MOV(0,Index_Write_Control)OTL(Update_Archive);
   62: NOP();
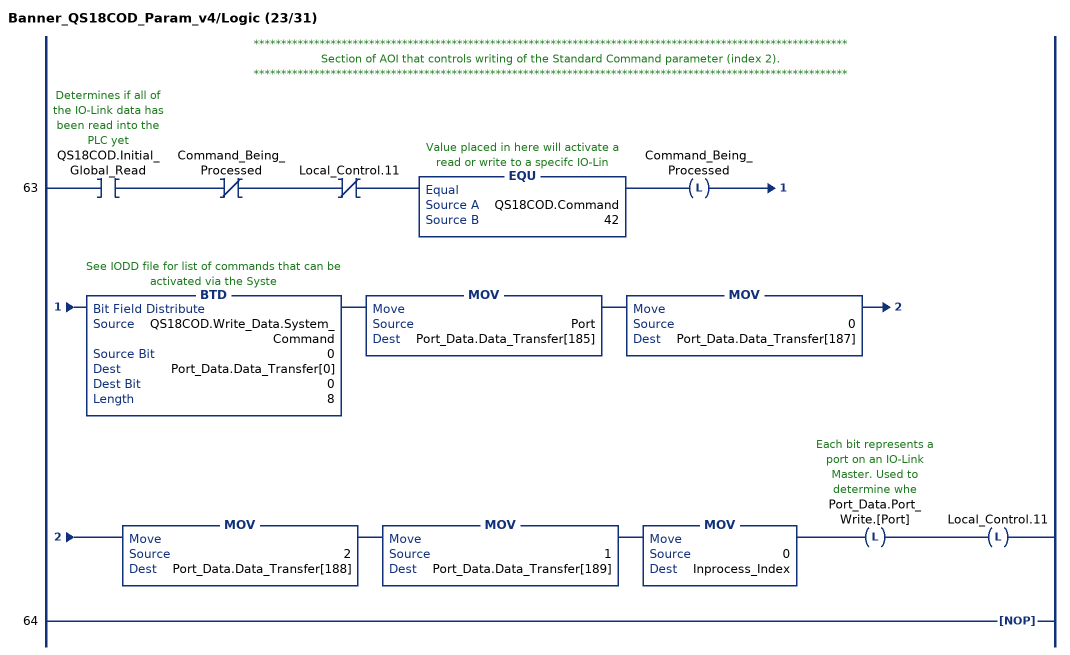
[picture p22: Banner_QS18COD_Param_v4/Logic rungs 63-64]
   // ************************************************************************************************************
   // Section of AOI that controls writing of the Standard Command parameter (index 2).
   // ************************************************************************************************************
   63: XIC(QS18COD.Initial_Global_Read)XIO(Command_Being_Processed)XIO(Local_Control.11)EQU(QS18COD.Command,42)OTL(Command_Being_Processed)BTD(QS18COD.Write_Data.System_Command,0,Port_Data.Data_Transfer[0],0,8)MOV(Port,Port_Data.Data_Transfer[185])MOV(0,Port_Data.Data_Transfer[187])MOV(2,Port_Data.Data_Transfer[188])MOV(1,Port_Data.Data_Transfer[189])MOV(0,Inprocess_Index)OTL(Port_Data.Port_Write.[Port])OTL(Local_Control.11);
   64: NOP();
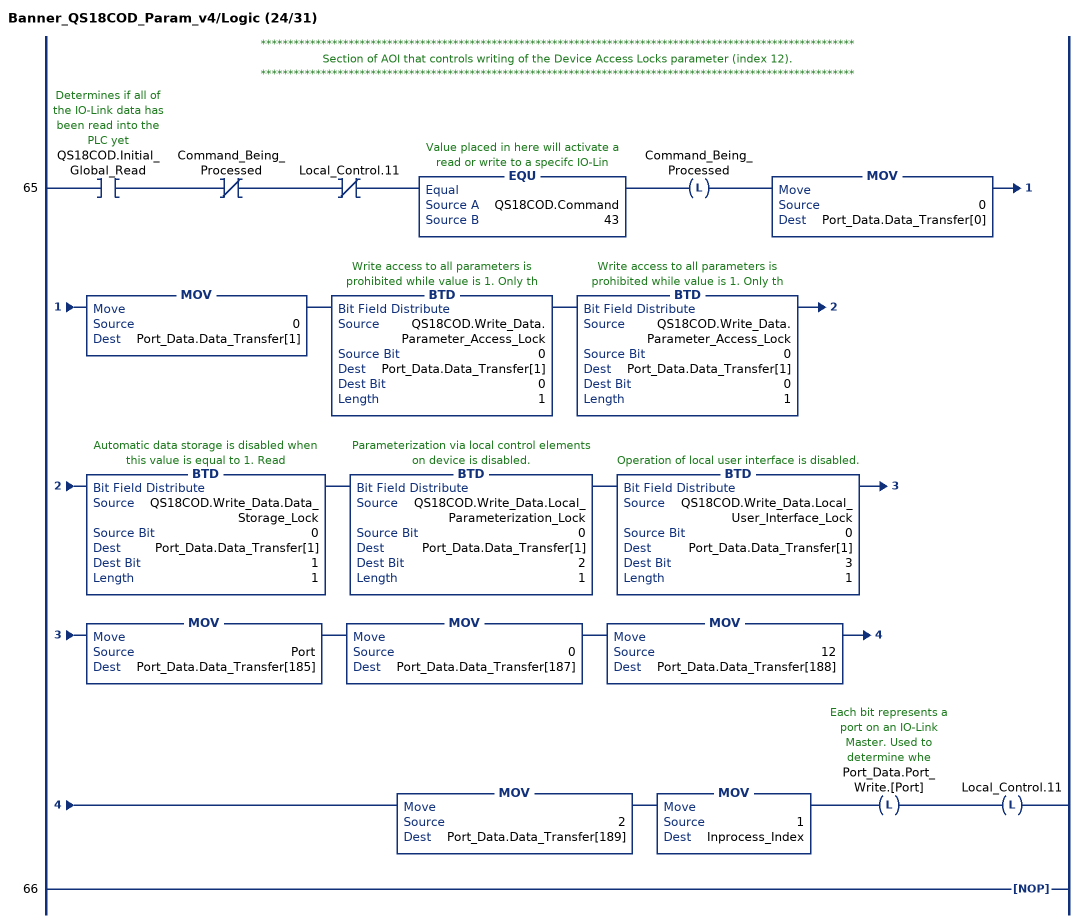
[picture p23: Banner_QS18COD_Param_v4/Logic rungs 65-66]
   // ************************************************************************************************************
   // Section of AOI that controls writing of the Device Access Locks parameter (index 12).
   // ************************************************************************************************************
   65: XIC(QS18COD.Initial_Global_Read)XIO(Command_Being_Processed)XIO(Local_Control.11)EQU(QS18COD.Command,43)OTL(Command_Being_Processed)MOV(0,Port_Data.Data_Transfer[0])MOV(0,Port_Data.Data_Transfer[1])BTD(QS18COD.Write_Data.Parameter_Access_Lock,0,Port_Data.Data_Transfer[1],0,1)BTD(QS18COD.Write_Data.Parameter_Access_Lock,0,Port_Data.Data_Transfer[1],0,1)BTD(QS18COD.Write_Data.Data_Storage_Lock,0,Port_Data.Data_Transfer[1],1,1)BTD(QS18COD.Write_Data.Local_Parameterization_Lock,0,Port_Data.Data_Transfer[1],2,1)BTD(QS18COD.Write_Data.Local_User_Interface_Lock,0,Port_Data.Data_Transfer[1],3,1)MOV(Port,Port_Data.Data_Transfer[185])MOV(0,Port_Data.Data_Transfer[187])MOV(12,Port_Data.Data_Transfer[188])MOV(2,Port_Data.Data_Transfer[189])MOV(1,Inprocess_Index)OTL(Port_Data.Port_Write.[Port])OTL(Local_Control.11);
   66: NOP();
